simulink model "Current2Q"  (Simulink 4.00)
settings: Solver=ode45  StartTime=0.0  StopTime=0.1  MaxStep=0.000005  RelTol=1e-3
undefined symbols (not defined in the file or in its folder): di, La, Ra, Ts, Ttc, Udc
libraries: simulink3 x1

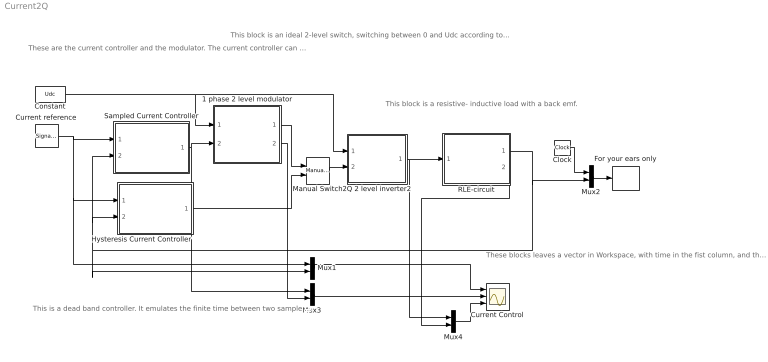
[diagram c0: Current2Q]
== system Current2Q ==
  note: These are the current controller and the modulator. The current controller can emulate several types of controllers.The most didactic is the "fast" but the most realistic is the "slow" and the "slow with Smith Predictor".
  note: This is a dead band controller. It emulates the finite time between two sample time instants, and a dead band.
  note: This block is an ideal 2-level switch, switching between 0 and Udc according to the input signal .
  note: This block is a resistive- inductive load with a back emf.
  note: These blocks leaves a vector in Workspace, with time in the fist column, and the current in the second. Use th file "Playsound" to listen to the sound of the converter, IF you have a sound card in your computer.
  1 phase 2 level modulator : Subsystem  mask{Random=Fixed frequency, Ts=Ts}
      mask prompts: Random "Fixed or random modulation?"; Ts "Sampling interval"
      mask help: Carrier Wave modulator that uses either fixed frequency modulation or random modulation. The fixed frequency modulation uses 1/(2Ts) as modulation frequency. The random modulation selects the modulatio frequency by random every sampling instant. The selection uses either 1/Ts, 1/(2Ts) or 1/(3Ts) as carrier wave frequency.
  2Q 2 level inverter2 : Subsystem
  Clock : Clock
  Constant : Constant  Value=Udc
  Current reference : SignalGenerator  WaveForm=square  Amplitude=5  Frequency=20  Units=Hertz
  Current Control : Scope  NumInputPorts=3
  For your ears only : ToWorkspace  VariableName=snd  SampleTime=-1  SaveFormat=Array
  Hysteresis Current Controller : Subsystem
  Manual Switch : simulink3/Nonlinear/Manual Switch  sw=1  action=0
  Mux{1..4} (4 alike) : Mux  Inputs=2
  RLE-circuit : Subsystem  mask(RLE-circuit){L=La, R=Ra, e0=40, i0=0}
      mask prompts: L "L [H]"; R "R [ohm]"; e0 "Back emf"; i0 "Starting Current"
      mask help: Parametrar
  Sampled Current Controller : Subsystem  mask{R=Ra, L=La, Kp=(La/Ttc+Ra/2), Ti=La/Ra+Ttc/2, Ttc=Ts, Umax=Udc, Umin=0, e0=40, SlowFast=Fast computer}
      mask prompts: R "Load resistance"; L "Load inductance"; Kp "Controller gain"; Ti "Integral Time Constant"; Ttc "Sampling time [s]"; Umax "Max output signal"; Umin "Min output signal"; e0 "Starting emf"; SlowFast "Controller type"
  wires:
  RLE-circuit/1(i) -> Hysteresis Current Controller/2(Act), Sampled Current Controller/2(Act), Mux1/2, Mux2/2
  Constant/1 -> 2Q 2 level inverter2/1(Udc), 1 phase 2 level modulator/1(Udc)
  2Q 2 level inverter2/1(v) -> RLE-circuit/1(u), Mux4/1
  Clock/1 -> Mux2/1
  Mux2/1 -> For your ears only/1
  Sampled Current Controller/1(u*) -> 1 phase 2 level modulator/2(va*), Mux3/1
  Mux1/1 -> Current Control/1
  Mux3/1 -> Current Control/2
  Current reference/1 -> Hysteresis Current Controller/1(Ref), Mux1/1, Sampled Current Controller/1(Ref)
  1 phase 2 level modulator/1(sa) -> Manual Switch/1
  Hysteresis Current Controller/1(s) -> Manual Switch/2
  Manual Switch/1 -> 2Q 2 level inverter2/2(s)
  1 phase 2 level modulator/2(um) -> Mux3/2
  RLE-circuit/2(" e") -> Mux4/2
  Mux4/1 -> Current Control/3

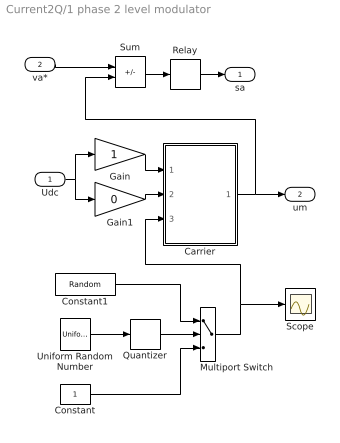
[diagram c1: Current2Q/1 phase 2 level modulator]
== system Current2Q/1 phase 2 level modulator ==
  Udc : Inport  Port=1  LatchInput=off
  va* : Inport  Port=2  LatchInput=off
  Carrier : Subsystem
  Constant : Constant  Value=1
  Constant1 : Constant  Value=Random
  Gain : Gain  Gain=1  Multiplication=Element-wise(K.*u)  SaturateOnIntegerOverflow=on
  Gain1 : Gain  Gain=0  Multiplication=Element-wise(K.*u)  SaturateOnIntegerOverflow=on
  Multiport Switch : MultiPortSwitch  Inputs=2
  Quantizer : Quantizer  QuantizationInterval=1  LinearizeAsGain=on
  Relay : Relay  OnSwitchValue=eps  OffSwitchValue=eps  OnOutputValue=1  OffOutputValue=-1
  Scope : Scope
  Sum : Sum  Inputs=+-  SaturateOnIntegerOverflow=on
  Uniform Random Number : UniformRandomNumber  Minimum=1  Maximum=3  Seed=0.9874  SampleTime=Ts
  sa : Outport  Port=1  InitialOutput=0
  um : Outport  Port=2  InitialOutput=0
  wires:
  Carrier/1(um) -> um/1, Sum/2
  Gain1/1 -> Carrier/2(Umin)
  Gain/1 -> Carrier/1(Umax)
  Udc/1 -> Gain1/1, Gain/1
  Relay/1 -> sa/1
  Sum/1 -> Relay/1
  va*/1 -> Sum/1
  Quantizer/1 -> Multiport Switch/2
  Uniform Random Number/1 -> Quantizer/1
  Constant/1 -> Multiport Switch/3
  Multiport Switch/1 -> Carrier/3(x), Scope/1
  Constant1/1 -> Multiport Switch/1

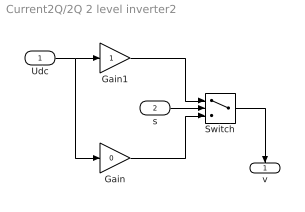
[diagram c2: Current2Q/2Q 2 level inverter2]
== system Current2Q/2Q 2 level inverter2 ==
  Udc : Inport  Port=1  LatchInput=off
  s : Inport  Port=2  LatchInput=off
  Gain : Gain  Gain=0  Multiplication=Element-wise(K.*u)  SaturateOnIntegerOverflow=on
  Gain1 : Gain  Gain=1  Multiplication=Element-wise(K.*u)  SaturateOnIntegerOverflow=on
  Switch : Switch  Threshold=0
  v : Outport  Orientation=down  Port=1  InitialOutput=0
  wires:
  Udc/1 -> Gain/1, Gain1/1
  Switch/1 -> v/1
  s/1 -> Switch/2
  Gain/1 -> Switch/3
  Gain1/1 -> Switch/1

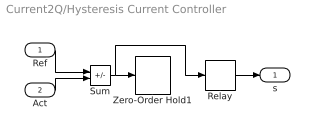
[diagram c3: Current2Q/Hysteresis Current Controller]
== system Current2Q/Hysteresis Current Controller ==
  Ref : Inport  Port=1  LatchInput=off
  Act : Inport  Port=2  LatchInput=off
  Relay : Relay  OnSwitchValue=di/2  OffSwitchValue=-di/2  OnOutputValue=1  OffOutputValue=-1
  Sum : Sum  Inputs=+-  SaturateOnIntegerOverflow=on
  Zero-Order Hold1 : ZeroOrderHold  SampleTime=Ts/4
  s : Outport  Port=1
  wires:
  Sum/1 -> Zero-Order Hold1/1, Relay/1
  Ref/1 -> Sum/1
  Act/1 -> Sum/2
  Relay/1 -> s/1

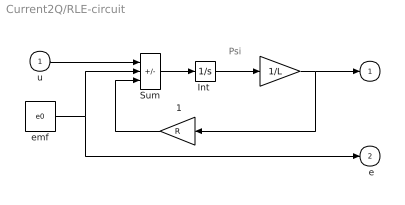
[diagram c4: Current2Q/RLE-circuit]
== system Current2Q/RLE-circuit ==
  note: i
  note: Psi
  u : Inport  Port=1  LatchInput=off
  " " : Gain  Gain=1/L  Multiplication=Element-wise(K.*u)  SaturateOnIntegerOverflow=on
  " 1" : Gain  Orientation=left  Gain=R  Multiplication=Element-wise(K.*u)  SaturateOnIntegerOverflow=on
  "Int " : Integrator  ExternalReset=none  InitialConditionSource=internal  InitialCondition=i0*L  LimitOutput=off  UpperSaturationLimit=inf  LowerSaturationLimit=-inf  ShowSaturationPort=off  ShowStatePort=off  AbsoluteTolerance=auto
  Sum : Sum  Inputs=+--  SaturateOnIntegerOverflow=on
  emf : Constant  Value=e0
  i : Outport  Port=1  InitialOutput=0
  " e" : Outport  Port=2  InitialOutput=0
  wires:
  " "/1 -> i/1, " 1"/1
  " 1"/1 -> Sum/3
  u/1 -> Sum/1
  Sum/1 -> "Int "/1
  "Int "/1 -> " "/1
  emf/1 -> Sum/2, " e"/1

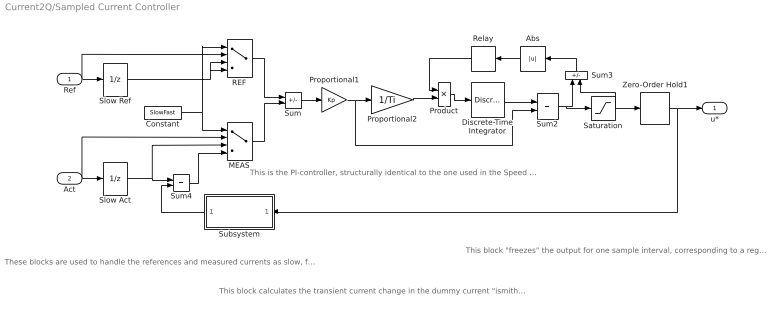
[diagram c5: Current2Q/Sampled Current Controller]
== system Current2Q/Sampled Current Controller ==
  note: These blocks are used to handle the references and measured currents as slow, fast or fast computer with Smith predictor.
  note: This block calculates the transient current change in the dummy current "ismith" The smith predictor calculates the current change that would have been measured if the computer was "fast", i.e. without the delay that a slow computer has. The calculated current change equals the real current change, but informing the controller one sampling interval earlier, thus allowing a high (deadbeat) gain.
  note: This is the PI-controller, structurally identical to the one used in the Speed Controller
  note: This block "freezes" the output for one sample interval, corresponding to a register in a microcontroller where the reference voltages are written once every sampling inteval.
  Ref : Inport  Port=1  LatchInput=off
  Act : Inport  Port=2  LatchInput=off
  Abs : Abs  Orientation=left  SaturateOnIntegerOverflow=on
  Constant : Constant  Value=SlowFast
  Discrete-Time Integrator : DiscreteIntegrator  IntegratorMethod=ForwardEuler  ExternalReset=none  InitialConditionSource=internal  InitialCondition=e0  LimitOutput=on  UpperSaturationLimit=Umax  LowerSaturationLimit=Umin  ShowSaturationPort=off  ShowStatePort=off  SampleTime=Ttc
  MEAS : MultiPortSwitch  Inputs=3
  Product : Product  Inputs=2  Multiplication=Element-wise(.*)  SaturateOnIntegerOverflow=on
  Proportional1 : Gain  Gain=Kp  Multiplication=Element-wise(K.*u)  SaturateOnIntegerOverflow=on
  Proportional2 : Gain  Gain=1/Ti  Multiplication=Element-wise(K.*u)  SaturateOnIntegerOverflow=on
  REF : MultiPortSwitch  Inputs=3
  Relay : Relay  Orientation=left  OnSwitchValue=eps  OffSwitchValue=eps  OnOutputValue=0  OffOutputValue=1
  Saturation : Saturate  UpperLimit=Umax  LowerLimit=Umin  LinearizeAsGain=on
  Slow Act : UnitDelay  X0=0  SampleTime=Ttc
  Slow Ref : UnitDelay  X0=0  SampleTime=Ttc
  Subsystem : Subsystem  Orientation=left
  Sum : Sum  Inputs=+-  SaturateOnIntegerOverflow=on
  Sum2 : Sum  Inputs=++  SaturateOnIntegerOverflow=on
  Sum3 : Sum  Orientation=up  Inputs=+-  SaturateOnIntegerOverflow=on
  Sum4 : Sum  Inputs=++  SaturateOnIntegerOverflow=on
  Zero-Order Hold1 : ZeroOrderHold  SampleTime=Ttc
  u* : Outport  Port=1
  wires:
  Discrete-Time Integrator/1 -> Sum2/1
  Proportional1/1 -> Proportional2/1, Sum2/2
  Sum/1 -> Proportional1/1
  Sum2/1 -> Saturation/1, Sum3/1
  Saturation/1 -> Zero-Order Hold1/1, Sum3/2
  Proportional2/1 -> Product/2
  Product/1 -> Discrete-Time Integrator/1
  Relay/1 -> Product/1
  Ref/1 -> REF/2, Slow Ref/1
  Zero-Order Hold1/1 -> u*/1, Subsystem/1(u)
  Act/1 -> MEAS/2, Slow Act/1
  Slow Act/1 -> Sum4/1, MEAS/3
  Subsystem/1(di_smith) -> Sum4/2
  Constant/1 -> MEAS/1, REF/1
  Slow Ref/1 -> REF/3, REF/4
  REF/1 -> Sum/1
  Sum4/1 -> MEAS/4
  MEAS/1 -> Sum/2
  Sum3/1 -> Abs/1
  Abs/1 -> Relay/1

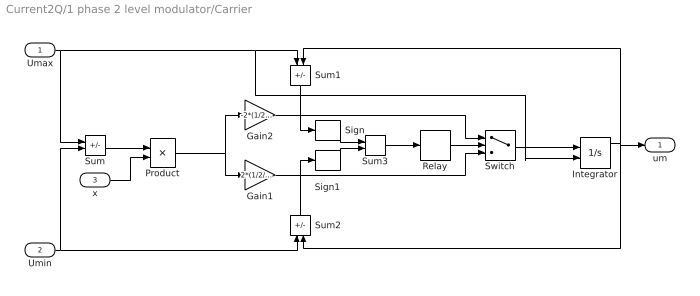
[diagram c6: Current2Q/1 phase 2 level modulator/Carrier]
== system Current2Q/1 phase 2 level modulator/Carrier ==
  Umax : Inport  Port=1  LatchInput=off
  Umin : Inport  Port=2  LatchInput=off
  x : Inport  Port=3  LatchInput=off
  Gain1 : Gain  Gain=2*(1/2/Ts)  Multiplication=Element-wise(K.*u)  SaturateOnIntegerOverflow=on
  Gain2 : Gain  Gain=-2*(1/2/Ts)  Multiplication=Element-wise(K.*u)  SaturateOnIntegerOverflow=on
  Integrator : Integrator  ExternalReset=none  InitialConditionSource=external  InitialCondition=0  LimitOutput=off  UpperSaturationLimit=inf  LowerSaturationLimit=-inf  ShowSaturationPort=off  ShowStatePort=off  AbsoluteTolerance=auto
  Product : Product  Inputs=2  Multiplication=Element-wise(.*)  SaturateOnIntegerOverflow=on
  Relay : Relay  OnSwitchValue=1  OffSwitchValue=-1  OnOutputValue=1  OffOutputValue=-1
  Sign : Signum
  Sign1 : Signum
  Sum : Sum  Inputs=+-  SaturateOnIntegerOverflow=on
  Sum1 : Sum  Orientation=down  Inputs=-+  SaturateOnIntegerOverflow=on
  Sum2 : Sum  Orientation=up  Inputs=-+  SaturateOnIntegerOverflow=on
  Sum3 : Sum  Inputs=++  SaturateOnIntegerOverflow=on
  Switch : Switch  Threshold=0
  um : Outport  Port=1
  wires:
  Switch/1 -> Integrator/1
  Umax/1 -> Sum/1, Sum1/1, Integrator/2
  Umin/1 -> Sum/2, Sum2/1
  Gain2/1 -> Switch/1
  Gain1/1 -> Switch/3
  Integrator/1 -> Sum1/2, um/1, Sum2/2
  Sum1/1 -> Sign/1
  Sum2/1 -> Sign1/1
  Sign/1 -> Sum3/1
  Sign1/1 -> Sum3/2
  Sum3/1 -> Relay/1
  Relay/1 -> Switch/2
  Sum/1 -> Product/1
  Product/1 -> Gain2/1, Gain1/1
  x/1 -> Product/2

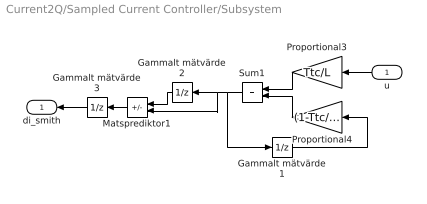
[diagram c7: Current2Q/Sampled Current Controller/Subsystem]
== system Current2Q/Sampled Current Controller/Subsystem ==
  u : Inport  Orientation=left  Port=1  LatchInput=off
  Gammalt mätvärde1 : UnitDelay  X0=e0/R  SampleTime=Ttc
  Gammalt mätvärde2 : UnitDelay  Orientation=left  X0=0  SampleTime=Ttc
  Gammalt mätvärde3 : UnitDelay  Orientation=left  X0=e0/R  SampleTime=Ttc
  Matsprediktor1 : Sum  Orientation=left  Inputs=-+  SaturateOnIntegerOverflow=on
  Proportional3 : Gain  Orientation=left  Gain=Ttc/L  Multiplication=Element-wise(K.*u)  SaturateOnIntegerOverflow=on
  Proportional4 : Gain  Orientation=left  Gain=(1-Ttc/(L/R))  Multiplication=Element-wise(K.*u)  SaturateOnIntegerOverflow=on
  Sum1 : Sum  Orientation=left  Inputs=++  SaturateOnIntegerOverflow=on
  di_smith : Outport  Orientation=left  Port=1
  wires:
  Proportional3/1 -> Sum1/1
  Gammalt mätvärde1/1 -> Proportional4/1
  Proportional4/1 -> Sum1/2
  Sum1/1 -> Gammalt mätvärde1/1, Gammalt mätvärde2/1, Matsprediktor1/2
  u/1 -> Proportional3/1
  Gammalt mätvärde2/1 -> Matsprediktor1/1
  Matsprediktor1/1 -> Gammalt mätvärde3/1
  Gammalt mätvärde3/1 -> di_smith/1
